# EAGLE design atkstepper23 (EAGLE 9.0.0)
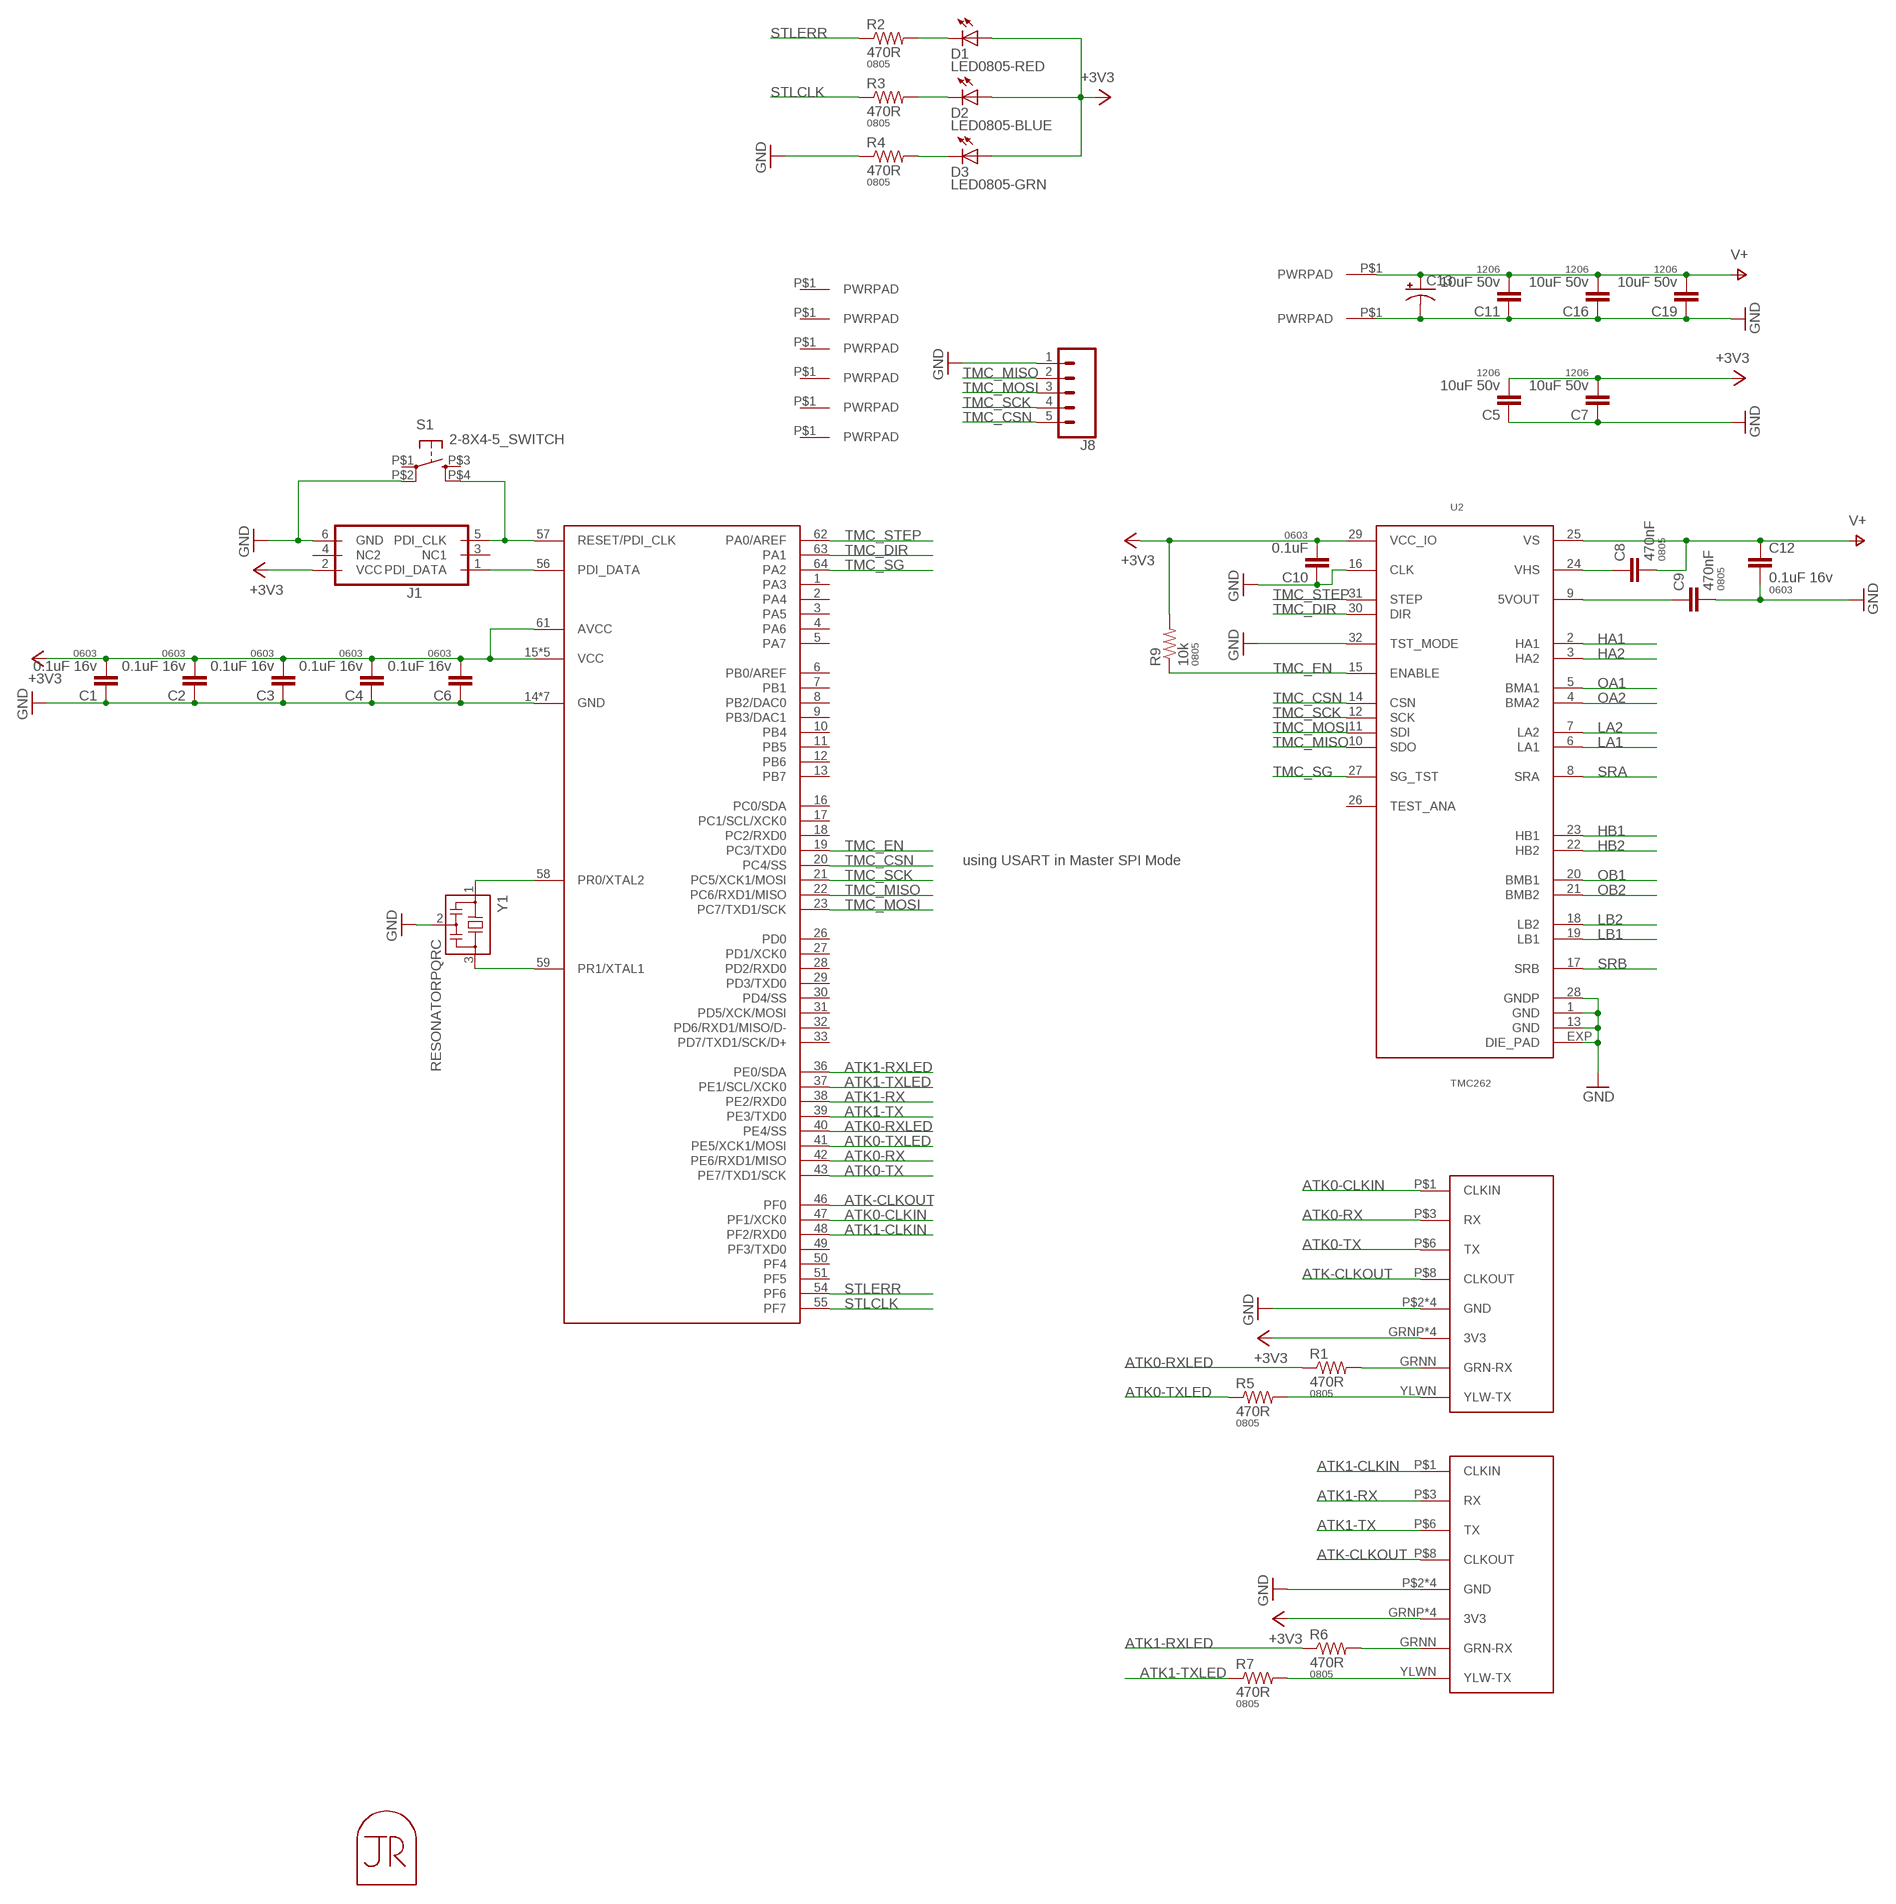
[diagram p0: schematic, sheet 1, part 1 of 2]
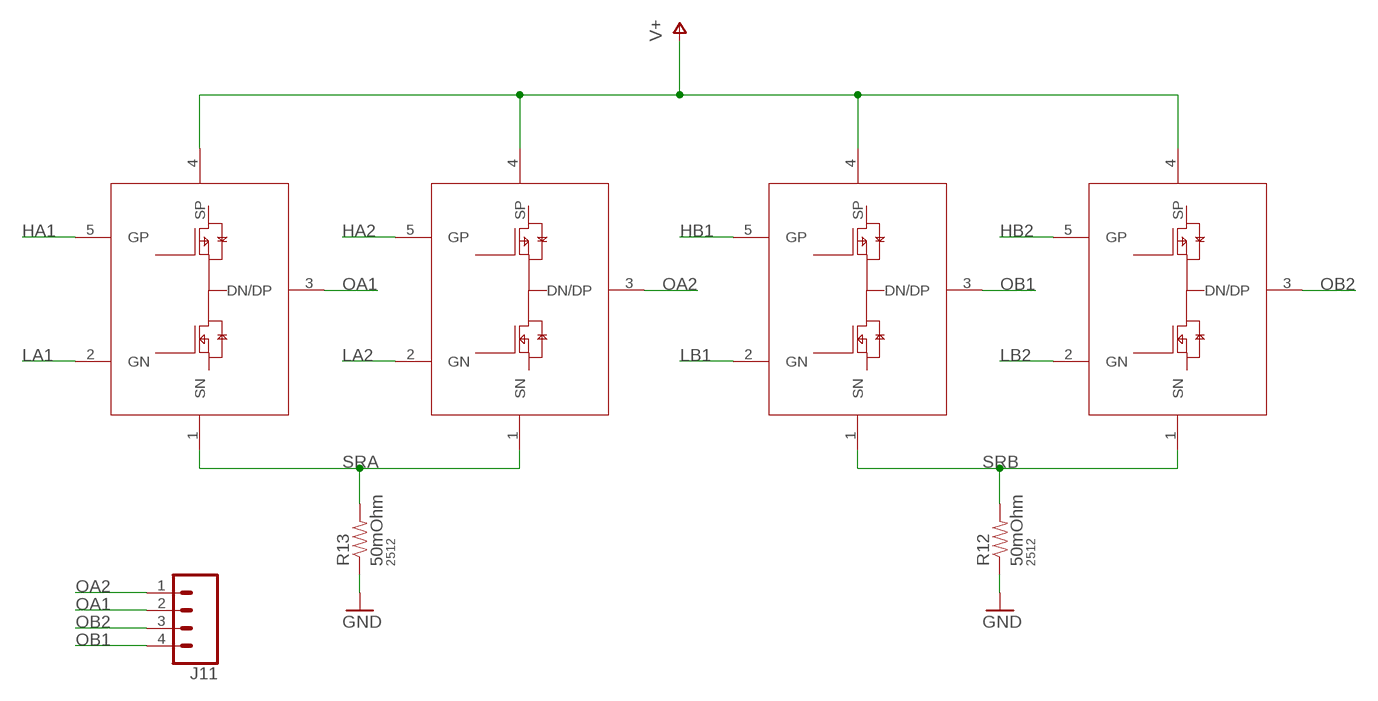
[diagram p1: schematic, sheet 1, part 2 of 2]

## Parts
C1  0.1uF 16v  CAP0603-CAP  [0603-CAP]
C2  0.1uF 16v  CAP0603-CAP  [0603-CAP]
C3  0.1uF 16v  CAP0603-CAP  [0603-CAP]
C4  0.1uF 16v  CAP0603-CAP  [0603-CAP]
C5  10uF 50v  CAP1206  [1206]
C6  0.1uF 16v  CAP0603-CAP  [0603-CAP]
C7  10uF 50v  CAP1206  [1206]
C8  470nF  CAP0805  [0805]
C9  470nF  CAP0805  [0805]
C10  0.1uF  CAP0603-CAP  [0603-CAP]
C11  10uF 50v  CAP1206  [1206]
C12  0.1uF 16v  CAP0603-CAP  [0603-CAP]
C13  CAP-POL-6.6X6.6  [6.6X6.6-CAP]
C16  10uF 50v  CAP1206  [1206]
C19  10uF 50v  CAP1206  [1206]
D1  LED0805-RED  LED0805  [LED0805]
D2  LED0805-BLUE  LED0805  [LED0805]
D3  LED0805-GRN  LED0805  [LED0805]
J1  PDIFEMALE_SMD  [PDI_2X3_SMD]
J2  ATK-PHY  [RJ45-LED-RJE7318800XXX]
J3  ATK-PHY  [RJ45-LED-RJE7318800XXX]
J4  PWRPADM3-SKINNY  [PWRPAD_3-25MM-SKINNY]
J5  PWRPADM3-SKINNY  [PWRPAD_3-25MM-SKINNY]
J6  PWRPADM3-SKINNY  [PWRPAD_3-25MM-SKINNY]
J7  PWRPADM3-SKINNY  [PWRPAD_3-25MM-SKINNY]
J8  CONN_05NO_SILK  [1X05_NO_SILK]
J9  PWRPAD  [PWRPAD_M3-PEM-MOUNT]
J10  PWRPAD  [PWRPAD_M3-PEM-MOUNT]
J11  CONN_04LONGPADS  [1X04_LONGPADS]
J12  PWRPADM3-SKINNY  [PWRPAD_3-25MM-SKINNY]
J13  PWRPADM3-SKINNY  [PWRPAD_3-25MM-SKINNY]
MP1  JRTOMBSTONE  [JRTOMBSTONE]
Q1  PNPAIR-FDD8424H  [DPAK-5]
Q2  PNPAIR-FDD8424H  [DPAK-5]
Q3  PNPAIR-FDD8424H  [DPAK-5]
Q4  PNPAIR-FDD8424H  [DPAK-5]
R1  470R  RESISTOR0805-RES  [0805]
R2  470R  RESISTOR0805-RES  [0805]
R3  470R  RESISTOR0805-RES  [0805]
R4  470R  RESISTOR0805-RES  [0805]
R5  470R  RESISTOR0805-RES  [0805]
R6  470R  RESISTOR0805-RES  [0805]
R7  470R  RESISTOR0805-RES  [0805]
R9  10k  RESISTOR0805-RES  [0805]
R12  50mOhm  RESISTOR2512  [R2512]
R13  50mOhm  RESISTOR2512  [R2512]
S1  2-8X4-5_SWITCH  [TACT-SWITCH-KMR6]
U1  ATXMEGA_A3UQFN  [QFN-64-9X9MM]
U2  TMC262  [QFN32]
Y1  RESONATORPQRC  [RES_PRQC]

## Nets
+3V3: C1.2 C2.2 C3.2 C4.2 C5.2 C6.2 C7.2 C10.2 D1.1(A) D2.1(A) D3.1(A) J1.2(VCC) J2.GRNP(3V3) J2.P$4(3V3) J2.P$5(3V3) J2.YLWP(3V3) J3.GRNP(3V3) J3.P$4(3V3) J3.P$5(3V3) J3.YLWP(3V3) R9.2 U1.15(VCC) U1.25(VCC) U1.35(VCC) U1.45(VCC) U1.53(VCC) U1.61(AVCC) U2.29(VCC_IO)
ATK0-CLKIN: J2.P$1(CLKIN) U1.47(PF1/XCK0)
ATK0-RX: J2.P$3(RX) U1.42(PE6/RXD1/MISO)
ATK0-RXLED: R1.1 U1.40(PE4/SS)
ATK0-TX: J2.P$6(TX) U1.43(PE7/TXD1/SCK)
ATK0-TXLED: R5.1 U1.41(PE5/XCK1/MOSI)
ATK1-CLKIN: J3.P$1(CLKIN) U1.48(PF2/RXD0)
ATK1-RX: J3.P$3(RX) U1.38(PE2/RXD0)
ATK1-RXLED: R6.1 U1.36(PE0/SDA)
ATK1-TX: J3.P$6(TX) U1.39(PE3/TXD0)
ATK1-TXLED: R7.1 U1.37(PE1/SCL/XCK0)
ATK-CLKOUT: J2.P$8(CLKOUT) J3.P$8(CLKOUT) U1.46(PF0)
GND: C1.1 C2.1 C3.1 C4.1 C5.1 C6.1 C7.1 C9.2 C10.1 C11.1 C12.2 C13.- C16.1 C19.1 J1.6(GND) J2.P$2(GND) J2.P$7(GND) J2.SHDL1(GND) J2.SHDL2(GND) J3.P$2(GND) J3.P$7(GND) J3.SHDL1(GND) J3.SHDL2(GND) J8.1 J10.P$1(PWRPAD) R4.1 R12.1 R13.1 S1.P$2(P1) U1.14(GND) U1.24(GND) U1.34(GND) U1.44(GND) U1.52(GND) U1.60(GND) U1.P$1(GND) U2.1(GND) U2.13(GND) U2.16(CLK) U2.28(GNDP) U2.32(TST_MODE) U2.EXP(DIE_PAD) Y1.2
HA1: Q1.5(GP) U2.2(HA1)
HA2: Q2.5(GP) U2.3(HA2)
HB1: Q3.5(GP) U2.23(HB1)
HB2: Q4.5(GP) U2.22(HB2)
LA1: Q1.2(GN) U2.6(LA1)
LA2: Q2.2(GN) U2.7(LA2)
LB1: Q3.2(GN) U2.19(LB1)
LB2: Q4.2(GN) U2.18(LB2)
N$1: D3.2(C) R4.2
N$2: C8.1 U2.24(VHS)
N$3: C9.1 U2.9(5VOUT)
N$4: J1.5(PDI_CLK) S1.P$4(S1) U1.57(RESET/PDI_CLK)
N$5: D2.2(C) R3.2
N$6: D1.2(C) R2.2
N$7: U1.58(PR0/XTAL2) Y1.1
N$8: U1.59(PR1/XTAL1) Y1.3
N$10: J1.1(PDI_DATA) U1.56(PDI_DATA)
N$11: J3.GRNN(GRN-RX) R6.2
N$12: J3.YLWN(YLW-TX) R7.2
N$17: J2.GRNN(GRN-RX) R1.2
N$18: J2.YLWN(YLW-TX) R5.2
OA1: J11.2 Q1.3(DN/DP) U2.5(BMA1)
OA2: J11.1 Q2.3(DN/DP) U2.4(BMA2)
OB1: J11.4 Q3.3(DN/DP) U2.20(BMB1)
OB2: J11.3 Q4.3(DN/DP) U2.21(BMB2)
SRA: Q1.1(SN) Q2.1(SN) R13.2 U2.8(SRA)
SRB: Q3.1(SN) Q4.1(SN) R12.2 U2.17(SRB)
STLCLK: R3.1 U1.55(PF7)
STLERR: R2.1 U1.54(PF6)
TMC_CSN: J8.5 U1.20(PC4/SS) U2.14(CSN)
TMC_DIR: U1.63(PA1) U2.30(DIR)
TMC_EN: R9.1 U1.19(PC3/TXD0) U2.15(ENABLE)
TMC_MISO: J8.2 U1.22(PC6/RXD1/MISO) U2.10(SDO)
TMC_MOSI: J8.3 U1.23(PC7/TXD1/SCK) U2.11(SDI)
TMC_SCK: J8.4 U1.21(PC5/XCK1/MOSI) U2.12(SCK)
TMC_SG: U1.64(PA2) U2.27(SG_TST)
TMC_STEP: U1.62(PA0/AREF) U2.31(STEP)
V+: C8.2 C11.2 C12.1 C13.+ C16.2 C19.2 J9.P$1(PWRPAD) Q1.4(SP) Q2.4(SP) Q3.4(SP) Q4.4(SP) U2.25(VS)
Unconnected: J1.3(NC1) J1.4(NC2) J4.P$1(PWRPAD) J5.P$1(PWRPAD) J6.P$1(PWRPAD) J7.P$1(PWRPAD) J12.P$1(PWRPAD) J13.P$1(PWRPAD) S1.P$1(P) S1.P$3(S) U1.1(PA3) U1.2(PA4) U1.3(PA5) U1.4(PA6) U1.5(PA7) U1.6(PB0/AREF) U1.7(PB1) U1.8(PB2/DAC0) U1.9(PB3/DAC1) U1.10(PB4) U1.11(PB5) U1.12(PB6) U1.13(PB7) U1.16(PC0/SDA) U1.17(PC1/SCL/XCK0) U1.18(PC2/RXD0) U1.26(PD0) U1.27(PD1/XCK0) U1.28(PD2/RXD0) U1.29(PD3/TXD0) U1.30(PD4/SS) U1.31(PD5/XCK/MOSI) U1.32(PD6/RXD1/MISO/D-) U1.33(PD7/TXD1/SCK/D+) U1.49(PF3/TXD0) U1.50(PF4) U1.51(PF5) U2.26(TEST_ANA)

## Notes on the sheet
- using USART in Master SPI Mode

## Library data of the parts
C1-C4 C6 C10 C12 = borkedlabs-passives:CAP: Capacitor; PACKAGE: 0603
C5 C7 C11 C16 C19 = borkedlabs-passives:CAP: Capacitor; PACKAGE: 1206
C8 C9 = borkedlabs-passives:CAP: Capacitor; PACKAGE: 0805
C13 = borkedlabs-passives:CAP-POL
D1-D3 = lights:LED: LED
J1 = microcontrollers:PDI: Multi connection point. Often used as Generic Header-pin footprint for 0.1 inch spaced/style header connections You can populate with any combo of single row headers, but if you'd like an exact match, check these: Header - 2x3 (Male, 0.1") (PRT-12807) Header - 2x3 (Female, 0.1") (PRT-13010) 2x3 Pin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; PROD_ID: CONN-11290
J2 J3 = connector:ATK-PHY
J4-J7 J9 J10 J12 J13 = power:PWRPAD
J8 = SparkFun-Connectors:CONN_05: Multi connection point. Often used as Generic Header-pin footprint for 0.1 inch spaced/style header connections On any of the 0.1 inch spaced packages, you can populate with these: Break Away Headers - Straight (PRT-00116) Break Away Male Headers - Right Angle (PRT-00553) Female Headers (PRT-00115)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
J11 = SparkFun-Connectors:CONN_04: Multi connection point. Often used as Generic Header-pin footprint for 0.1 inch spaced/style header connections On any of the 0.1 inch spaced packages, you can populate with these: Break Away Headers - Straight (PRT-00116) Break Away Male Headers - Right Angle (PRT-00553) Female Headers (PRT-00115)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; PROD_ID: CONN-09696
MP1 = connector:JRTOMBSTONE
Q1-Q4 = power:PNPAIR-FDD8424H
R1-R7 R9 = borkedlabs-passives:RESISTOR: Resistor; PACKAGE: 0805
R12 R13 = borkedlabs-passives:RESISTOR: Resistor; PACKAGE: 2512
S1 = fab:2-8X4-5_SWITCH
U1 = microcontrollers:ATXMEGA_A3U
U2 = power:TMC262
Y1 = passives:RESONATOR

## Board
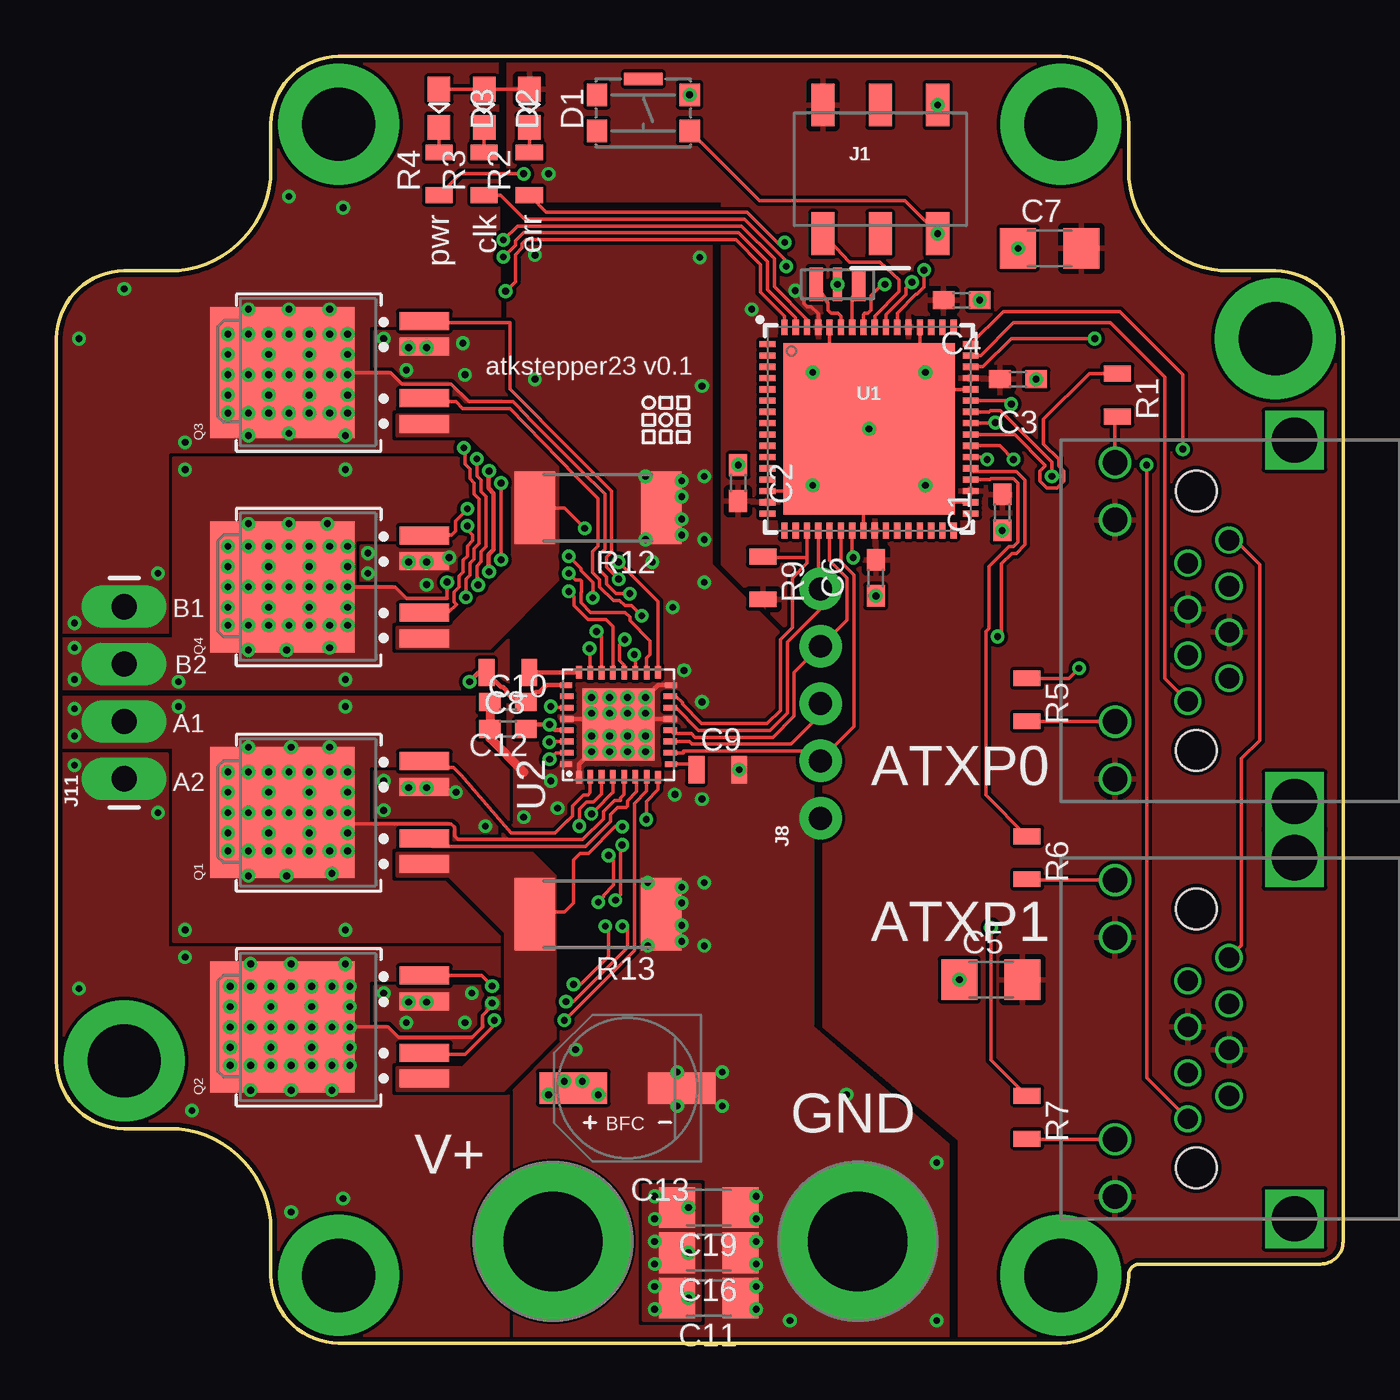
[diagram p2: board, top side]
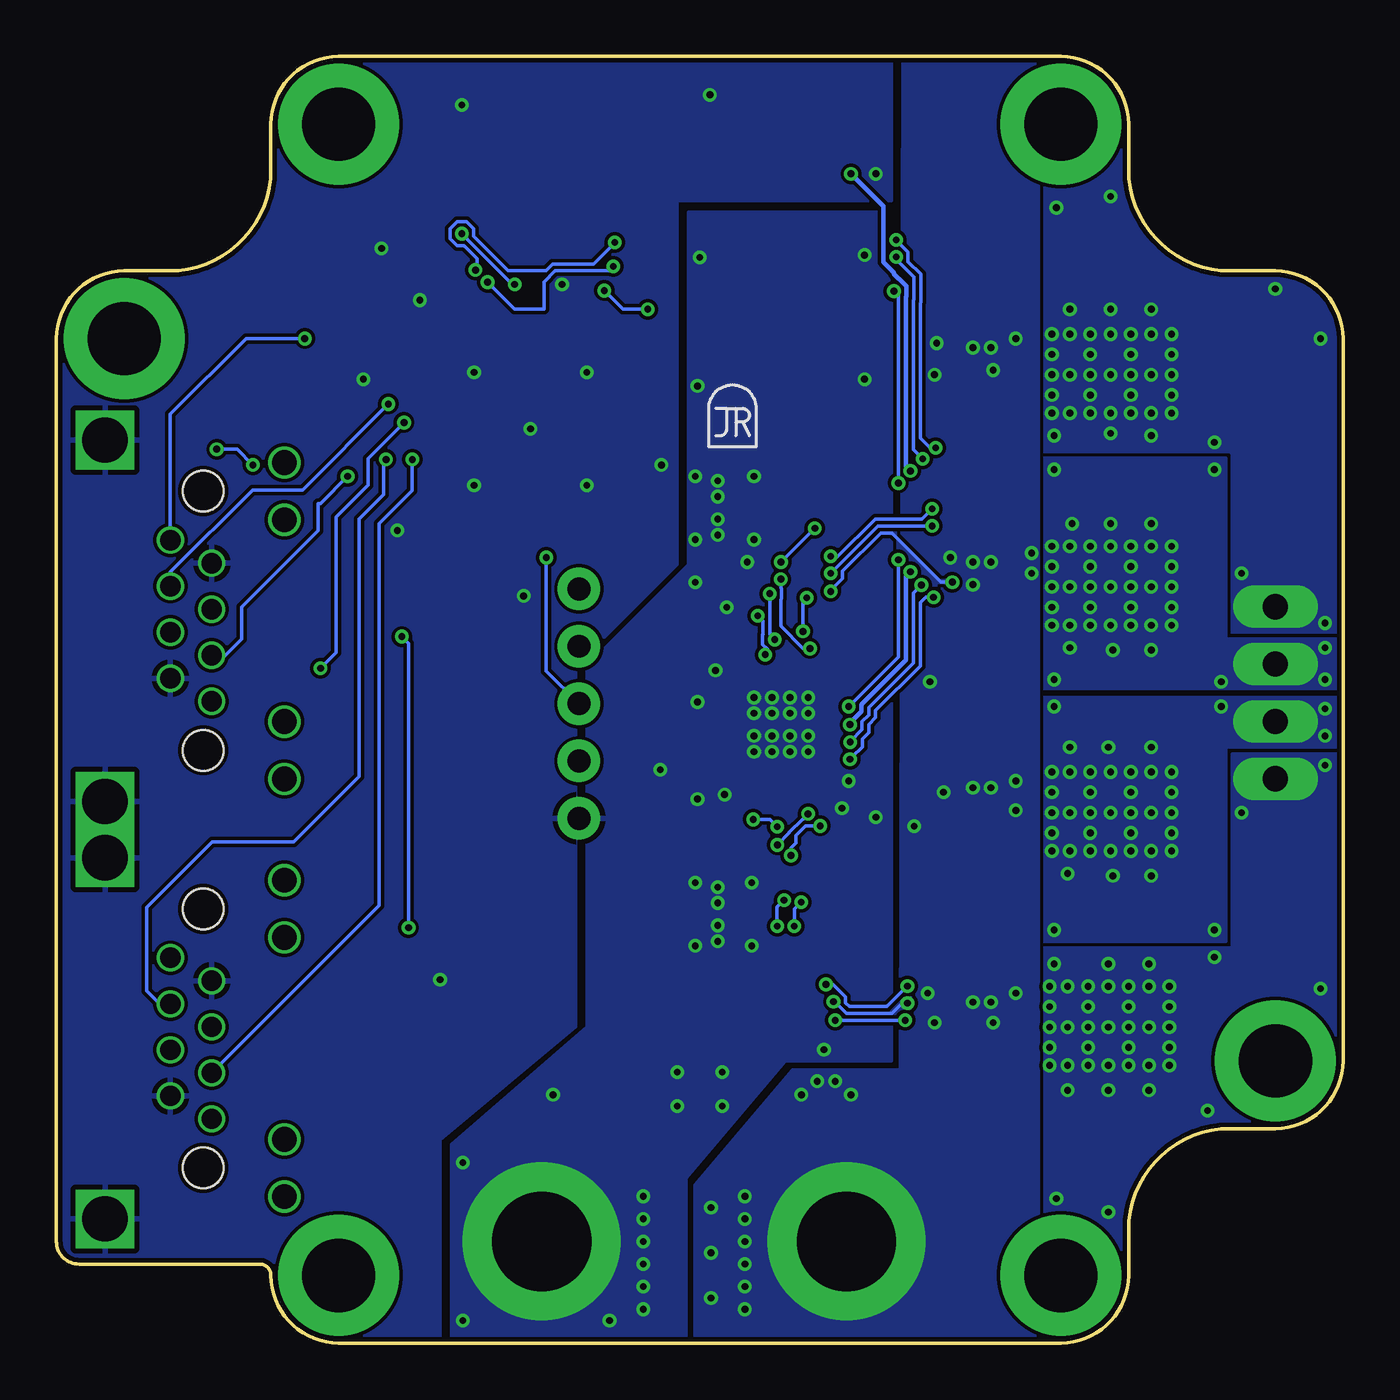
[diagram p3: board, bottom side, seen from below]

Size 57 x 57 mm. Coordinates in mm from the lower left corner, seen from the top.
Outline: 44.5,0 12.5,0 arc-90 9.5,3 9.5,5 arc90 5,9.5 3,9.5 arc-90 0,12.5 0,44.5 arc-90 3,47.5 5,47.5 arc90 9.5,52 9.5,54 arc-90 12.5,57 44.5,57 arc-90 47.5,54 47.5,52 arc90 52,47.5 54,47.5 arc-90 57,44.5 57,4.5 arc-90 56,3.5 48,3.5 arc90 47.5,3 arc-90 44.5,0
Copper layers (1*16): Top 0.035mm / dielectric 1.5mm / Bottom 0.035mm
Design rules "default *": minimum track width 6mil, minimum drill 0.3mm, track to track 6mil, track to pad 6mil, pad to pad 6mil, via to via 6mil, smd to smd 6mil, copper to edge 8mil, drill to drill 8mil, minimum pad ring 6mil, minimum via ring 6mil, stop-mask expansion 4mil, vias tented up to drill 27mil, thermal gap 9mil

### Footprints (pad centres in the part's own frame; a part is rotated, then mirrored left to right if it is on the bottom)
0603-CAP = smd 0.96 x 0.8: 1 -0.8,0; 2 0.8,0
1206 = smd 1.6 x 1.8: 1 -1.4,0; 2 1.4,0
0805 = smd 0.7 x 1.2: 1 -0.95,0; 2 0.95,0
6.6X6.6-CAP = smd 3 x 1.4: + 2.4,0; - -2.4,0
LED0805 = smd 1.1 x 1: 1 -0.85,0; 2 0.85,0
PDI_2X3_SMD = smd 1.02 x 1.9: 1 -2.54,-2.85; 2 -2.54,2.85; 3 0,-2.85; 4 0,2.85; 5 2.54,-2.85; 6 2.54,2.85
RJ45-LED-RJE7318800XXX = drill 1.1: GRNN 7.01,3.6; GRNP 4.47,3.6; YLWN -4.47,3.6; YLWP -7.01,3.6 | drill 0.9: P$1 -3.57,0.38; P$2 -2.55,-1.45; P$3 -1.53,0.38; P$4 -0.51,-1.45; P$5 0.51,0.38; P$6 1.53,-1.45; P$7 2.55,0.38; P$8 3.57,-1.45 | drill 2 square: SHDL1 -8,-4.35; SHDL2 8,-4.35 | hole 1.8: -5.74,0; 5.74,0
PWRPAD_3-25MM-SKINNY = drill 3.25 pad 5.35: P$1 0,0
1X05_NO_SILK = drill 1.016 pad 1.88: 1 0,0; 2 2.54,0; 3 5.08,0; 4 7.62,0; 5 10.16,0
PWRPAD_M3-PEM-MOUNT = drill 4.4 pad 7: P$1 0,0
1X04_LONGPADS = drill 1.118 pad 1.88 long: 1 0,0; 2 2.54,0; 3 5.08,0; 4 7.62,0
DPAK-5 = smd 0.8 x 2.2: 1 -2.28,-5.3; 2 -1.14,-5.3; 4 1.14,-5.3; 5 2.28,-5.3 | smd 5.8 x 6.4: 3 0,1
R2512 = smd 1.8 x 3.2: 1 -2.8,0; 2 2.8,0
TACT-SWITCH-KMR6 = smd 0.9 x 1: P$1 -2.05,0.8; P$2 2.05,0.8; P$3 -2.05,-0.8; P$4 2.05,-0.8 | smd 1.7 x 0.55: P$5 0,1.5
QFN-64-9X9MM = smd 0.7 x 0.275: 1 -4.5,3.75; 2 -4.5,3.25; 3 -4.5,2.75; 4 -4.5,2.25; 5 -4.5,1.75; 6 -4.5,1.25; 7 -4.5,0.75; 8 -4.5,0.25; 9 -4.5,-0.25; 10 -4.5,-0.75; 11 -4.5,-1.25; 12 -4.5,-1.75; 13 -4.5,-2.25; 14 -4.5,-2.75; 15 -4.5,-3.25; 16 -4.5,-3.75; 33 4.5,-3.75; 34 4.5,-3.25; 35 4.5,-2.75; 36 4.5,-2.25; 37 4.5,-1.75; 38 4.5,-1.25; 39 4.5,-0.75; 40 4.5,-0.25; 41 4.5,0.25; 42 4.5,0.75; 43 4.5,1.25; 44 4.5,1.75; 45 4.5,2.25; 46 4.5,2.75; 47 4.5,3.25; 48 4.5,3.75 | smd 0.275 x 0.7: 17 -3.75,-4.5; 18 -3.25,-4.5; 19 -2.75,-4.5; 20 -2.25,-4.5; 21 -1.75,-4.5; 22 -1.25,-4.5; 23 -0.75,-4.5; 24 -0.25,-4.5; 25 0.25,-4.5; 26 0.75,-4.5; 27 1.25,-4.5; 28 1.75,-4.5; 29 2.25,-4.5; 30 2.75,-4.5; 31 3.25,-4.5; 32 3.75,-4.5; 49 3.75,4.5; 50 3.25,4.5; 51 2.75,4.5; 52 2.25,4.5; 53 1.75,4.5; 54 1.25,4.5; 55 0.75,4.5; 56 0.25,4.5; 57 -0.25,4.5; 58 -0.75,4.5; 59 -1.25,4.5; 60 -1.75,4.5; 61 -2.25,4.5; 62 -2.75,4.5; 63 -3.25,4.5; 64 -3.75,4.5 | smd 7.6 x 7.6: P$1 0,0
QFN32 = smd 0.55 x 0.25: 1 -2.325,1.75; 8 -2.325,-1.75; 17 2.325,-1.75; 24 2.325,1.75 | smd 0.6 x 0.25: 2 -2.3,1.25; 3 -2.3,0.75; 4 -2.3,0.25; 5 -2.3,-0.25; 6 -2.3,-0.75; 7 -2.3,-1.25; 18 2.3,-1.25; 19 2.3,-0.75; 20 2.3,-0.25; 21 2.3,0.25; 22 2.3,0.75; 23 2.3,1.25 | smd 0.25 x 0.55: 9 -1.75,-2.325; 16 1.75,-2.325; 25 1.75,2.325; 32 -1.75,2.325 | smd 0.25 x 0.6: 10 -1.25,-2.3; 11 -0.75,-2.3; 12 -0.25,-2.3; 13 0.25,-2.3; 14 0.75,-2.3; 15 1.25,-2.3; 26 1.25,2.3; 27 0.75,2.3; 28 0.25,2.3; 29 -0.25,2.3; 30 -0.75,2.3; 31 -1.25,2.3 | smd 3.2 x 3.2: EXP 0,0
RES_PRQC = smd 0.6 x 1.5: 1 -0.95,0; 3 0.95,0 | smd 0.4 x 1.5: 2 0,0

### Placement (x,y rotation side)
C1  41.9,36.8 90 top
C2  30.2,38.1 270 top
C3  42.6,42.7 180 top
C4  40.1,46.2 180 top
C5  41.4,16.1 0 top
C6  36.3,33.9 90 top
C7  44,48.5 0 top
C8  20,29.7 180 top
C9  29.3,25.4 0 top
C10  20,27.2 0 top
C11  28.9,2 180 top
C12  20,28.4 180 top
C13  25.3,11.3 180 top
C16  28.9,4 180 top
C19  28.9,6 180 top
D1  20.95,54.7 270 top
D2  18.95,54.7 270 top
D3  16.95,54.7 270 top
J1  36.5,52 0 top
J2  50.5,32 90 top
J3  50.5,13.5 90 top
J4  12.5,3 180 top
J5  54,44.5 180 top
J6  44.5,3 180 top
J7  3,12.5 180 top
J8  33.85,23.25 90 top
J9  22,4.5 180 top
J10  35.5,4.5 180 top
J11  3,25 90 top
J12  12.5,54 180 top
J13  44.5,54 180 top
MP1  27,40.7 0 bottom
Q1  11,23.5 90 top
Q2  11,14 90 top
Q3  11,43 90 top
Q4  11,33.5 90 top
R1  47,42 270 top
R2  20.95,51.8 90 top
R3  18.95,51.8 90 top
R4  16.95,51.8 90 top
R5  43,28.5 270 top
R6  43,21.5 270 top
R7  43,10 270 top
R9  31.3,33.9 270 top
R12  24,37 180 top
R13  24,19 180 top
S1  26,54.5 0 top
U1  36,40.5 0 top
U2  24.9,27.4 90 top
U$5  [CBA-SILK-LOGO]  27,40.9 0 top
Y1  34.6,46.9 180 top

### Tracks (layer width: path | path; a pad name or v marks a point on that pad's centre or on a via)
+3V3  (via drill 0.3)
  Top 0.152: D1.1 D2.1 D3.1 | U1.61 33.75,45.6 33.43,45.92 33.26,45.92 33.12,46.05 33.12,46.23 v32.73,46.62
  Top 0.203: U2.29 22.09,27.15 v21.84,27.4 21,27.4 C10.2 | v19.16,34.16 19.16,34.45 19.14,34.47 19.14,34.93 19.37,35.16 19.37,37.64 19.14,37.87 19.14,38.33 19.16,38.35 v19.16,38.63
  Bottom 0.152: v32.73,46.62 31.9,45.8 v30.8,45.8
  Bottom 0.203: v21.84,27.4 21.84,27.47 21.34,27.97 21.34,28.29 19.37,30.26 19.37,33.96 v19.16,34.16 | v19.16,38.63 19.37,38.84 19.37,46.34 19.34,46.37 19.34,46.83 19.67,47.16 19.7,47.16 19.9,47.36 19.9,47.43 20.36,47.88 20.36,50.36 v21.8,51.8
  pour Top (rank 2): 20,58 20,50.6 29.5,50.6 29.5,34.5 34,30 34,14 40,9 40,-1 57.8,-0.8 57.8,58
ATK0-CLKIN
  Top 0.152: U1.47 40.95,43.75 42.4,45.2 46.7,45.2 49.1,42.8 49.1,29.45 J2.P$1
ATK0-RX  (via drill 0.3)
  Top 0.152: U1.42 41.32,41.25 41.38,41.31 41.82,41.31 44.1,39.03 v44.1,38.4
  Bottom 0.152: J2.P$3 49.53,30.47 48.8,31.2 48.8,32.6 45.4,36 45.4,37.2 45.3,37.2 v44.1,38.4
ATK0-RXLED
  Top 0.152: R1.1 45.75,42.95 43.73,40.93 43.73,39.83 44.41,39.16 44.41,38.85 44.63,38.62 44.63,38.18 44.32,37.87 43.88,37.87 43.57,38.18 43.57,38.62 43.8,38.85 43.8,38.91 42.45,40.25 U1.40
ATK0-TX  (via drill 0.3)
  Top 0.152: U1.43 42.15,41.75 v42.3,41.6
  Bottom 0.152: v42.3,41.6 46.1,37.8 48.3,37.8 51.95,34.15 J2.P$6
ATK0-TXLED  (via drill 0.3)
  Top 0.152: U1.41 41.57,40.75 v41.6,40.78 | v45.3,29.9 44.85,29.45 R5.1
  Bottom 0.152: v45.3,29.9 44.6,30.6 44.6,36.6 43.2,38 43.2,39.18 v41.6,40.78
ATK1-CLKIN  (via drill 0.3)
  Top 0.152: U1.48 41.95,45.7 47.1,45.7 49.9,42.9 v49.9,39.6 | v48.3,38.9 48.3,11.75 J3.P$1
  Bottom 0.152: v49.9,39.6 49,39.6 v48.3,38.9
ATK1-RX  (via drill 0.3)
  Top 0.152: U1.38 41.13,39.25 v41.24,39.14
  Bottom 0.152: v41.24,39.14 41.24,37.76 42.7,36.3 42.7,19.39 J3.P$3
ATK1-RXLED
  Top 0.152: U1.36 41.35,38.25 41.41,38.31 42.4,38.31 42.6,38.1 42.6,35.5 42.4,35.29 42.19,35.29 41.3,34.4 41.3,31.65 41.17,31.52 41.17,24.28 R6.1
ATK1-TX  (via drill 0.3)
  Top 0.152: U1.39 41.79,39.75 v42.4,39.14
  Bottom 0.152: v42.4,39.14 42.5,39.04 42.5,37.6 43.6,36.5 43.6,25.1 46.5,22.2 50.1,22.2 53,19.3 53,15.6 52.43,15.03 J3.P$6
ATK1-TXLED  (via drill 0.3)
  Top 0.152: U1.37 40.63,38.62 40.95,38.62 40.95,38.61 42.52,38.61 42.91,38.23 42.91,35.37 42.52,34.99 42.32,34.99 41.87,34.53 41.87,31.47 v41.7,31.3 | v41.4,18.4 41.4,12.55 R7.1
  Bottom 0.152: v41.7,31.3 41.4,31 v41.4,18.4
ATK-CLKOUT  (via drill 0.3)
  Top 0.152: U1.46 41.05,43.25 42.3,44.5 v46,44.5 | J2.P$8 52.23,35.57 53.3,34.5 53.3,26.7 52.5,25.9 52.5,17.62 J3.P$8
  Bottom 0.152: v46,44.5 48.6,44.5 51.95,41.15 J2.P$8
GND  (via drill 0.3)
  Top 0.152: R4.1 17.9,51.8 v20.7,51.8 | U1.60 34.25,42.25 35.9,40.6 | 35.9,40.6 U1.P$1 36.05,40.55 | U1.52 38.25,42.75 36.05,40.55 | U1.34 39.35,37.25 36.05,40.55 | U1.24 35.75,40.4 | 35.75,40.4 35.75,40.45 35.9,40.6 | U1.14 33.1,37.75 35.75,40.4 | U1.44 39.25,42.25 v38.5,43
  Top 0.203: U2.1 23.15,25.65 v23.7,26.2 | U2.13 26.35,27.65 v26.1,27.9 | U2.16 26.65,29.15 v26.1,28.6 | U2.28 23.45,27.65 v23.7,27.9
  Top 0.406: C12.2 C10.1 19.2,26.8 20.7,25.3
  other vias: 26.1,26.2 24.5,26.2 25.3,26.2 26.1,26.9 23.7,26.9 24.5,26.9 25.3,26.9 24.5,27.9 25.3,27.9 23.7,28.6 24.5,28.6 25.3,28.6 27.7,17.8 27.7,18.5 27.7,19.5 27.7,20.2 28.7,20.4 28.7,17.6 26.2,17.6 26.2,20.4 27.7,35.8 27.7,36.5 27.7,37.5 27.7,38.2 28.7,38.4 28.7,35.6 26.1,35.6 26.1,38.4 30.25,25.4 27.8,29.8 28.6,28.4 26.4,34.6 21.2,42.7 28.6,42.4 28.5,48.1 21.2,48.2 27.4,24.3 28.6,24.1 29.5,10.5 35,11 29.5,12 39,8 39,1 32.5,1 27.5,10.5 23,13 20.7,23.3 21.9,24.9 40.9,46.2 41.9,36 30.2,38.9 36.3,33.1 31,1.5 31,2.5 31,3.5 31,4.5 31,5.5 31,6.5 27.5,12 22.2,23.7 27.3,32.6 28.7,33.7 34.6,46.9 28.05,55.3 39.04,54.85 36,40.5 33.5,43 38.5,38 33.5,38 43.4,42.7 42.6,48.5 40,16.1
  pour Bottom: 29.1,-0.5 29.1,7.3 24.7,12.5 20,12.5 20,50.1 29,50.1 29,34.5 33.5,30 33.5,14 39.5,8.8 39.5,-0.5
  pour Top (no thermals): 25.8,35.3 29,35.3 29,38.7 25.8,38.7
  pour Top (no thermals): 25.8,17.3 29,17.3 29,20.7 25.8,20.7
  pour Bottom: 29.5,57.6 20,57.6 20,50.6 29.5,50.6 29.5,34.5 34,30 34,14 40,9 40,-0.5 57.5,-0.5 57.5,57.5
  pour Top (rank 6, no thermals): 39.5,-1 39.5,8.8 33.5,14 33.5,30 29,34.5 29,50.1 20,50.1 20,-1
HA1
  Top 0.152: Q1.5 16.58,25.5 17.6,25.5 17.93,25.17 20.13,22.61 22.1,22.61 22.64,23.14 22.64,23.13 22.86,23.36 22.86,23.79 23.36,24.28 23.54,24.28 23.65,24.39 U2.2
HA2  (via drill 0.3)
  Top 0.152: Q2.5 18.83,16.28 v19.3,15.81 | v22.91,15.89 23.23,15.89 24.47,17.13 24.47,18.31 v24.31,18.47 | v24.01,19.53 24.23,19.76 24.23,19.84 24.69,20.29 24.69,21.37 v24.46,21.6 | v23.17,22.91 23.17,23.66 23.48,23.98 23.8,23.98 24.15,24.32 U2.3
  Bottom 0.152: v19.3,15.81 20.2,14.91 21.87,14.91 22.04,15.08 22.04,15.35 22.59,15.89 v22.91,15.89 | v24.31,18.47 24.31,19.23 v24.01,19.53 | v24.46,21.6 24.46,21.94 24.23,22.16 24.23,22.48 23.81,22.91 v23.17,22.91
HB1  (via drill 0.3)
  Top 0.152: Q3.5 16.38,45.2 20.1,45.2 20.1,42.27 20.44,41.93 20.44,41.92 20.54,41.83 21.45,40.92 21.45,40.89 24.6,37.74 24.6,35.05 | v24.91,33.84 24.37,34.38 24.37,34.82 24.6,35.05 | 24.6,35.05 | U2.23 23.65,30.74 v23.62,30.77
  Bottom 0.152: v24.91,33.84 24.91,33.46 24.87,33.42 24.87,32.98 24.91,32.94 24.91,31.75 23.92,30.77 v23.62,30.77
HB2  (via drill 0.3)
  Top 0.152: Q4.5 16.32,35.8 17.5,35.8 17.67,35.97 17.67,36.42 v18.2,36.95 v18.2,36.96 | v22.7,34.86 v22.7,34.85 23.23,34.32 23.23,34.23 23.76,33.69 v23.76,33.02 | v23.93,31.53 24.15,31.31 U2.22
  Bottom 0.152: v18.2,36.96 18.66,36.51 20.73,36.51 22.42,34.82 22.66,34.82 v22.7,34.86 | v23.93,31.53 23.93,32.85 v23.76,33.02
LA1
  Top 0.152: U2.6 25.7,25.05 25.7,24.43 25.3,24.03 25.3,23.8 25.23,23.73 24.85,23.73 24.54,23.42 24.54,23.1 23.44,22 16.66,22 Q1.2
LA2  (via drill 0.3)
  Top 0.152: Q2.2 17.4,12.8 18.1,12.8 19.4,14.1 v19.4,14.3 | v22.5,14.3 25.6,17.4 25.6,23.9 26.15,24.45 U2.7
  Bottom 0.152: v19.4,14.3 v22.5,14.3
LB1  (via drill 0.3)
  Top 0.152: Q3.2 16.46,41.7 17.7,41.7 18,41.4 20.1,41.4 23,38.4 23.99,37.41 23.99,35.3 23.76,35.07 23.76,34.13 24.07,33.82 24.07,33.5 24.67,32.9 24.95,32.9 25.18,32.67 25.48,32.67 v25.93,32.22 | U2.19 25.65,30.45 v25.6,30.5
  Bottom 0.152: v25.6,30.5 25.5,30.6 25.5,30.74 25.71,30.95 25.71,31.39 25.7,31.4 25.7,31.99 v25.93,32.22
LB2  (via drill 0.3)
  Top 0.152: Q4.2 17.36,32.36 17.72,32.72 17.61,32.82 17.61,33.26 17.84,33.49 17.84,33.97 18.02,34.16 18.02,34.69 18.2,34.87 18.2,35.32 18.43,35.55 18.43,35.8 18.2,36.03 v18.2,36.2 | U2.18 26.15,30.35 26.3,30.5 26.3,31.1 25.4,32 25.4,32.16 25.2,32.36 23.67,32.36 23.23,32.8 23.23,33.24 23.26,33.27 23.26,33.76 23.23,33.8 23,33.8 v22.7,34.1
  Bottom 0.152: v18.2,36.2 20.6,36.2 v22.7,34.1
N$1
  Top 0.152: D3.2 R4.2
N$2
  Top 0.203: U2.24 23.12,29.7 C8.1
N$3
  Top 0.152: U2.9 28.35,25.65 C9.1
N$4  (via drill 0.3)
  Top 0.152: U1.57 35.75,45.57 35.8,45.62 35.95,45.62 36.08,45.76 36.08,46.4 36.58,46.9 v36.7,46.9 | S1.P$4 31.15,50.6 37.59,50.6 J1.5
  Bottom 0.152: J1.5 38.81,48.92 38.81,48.91 36.8,46.9 v36.7,46.9
  other vias: 39.04,49.15
N$5
  Top 0.152: D2.2 R3.2
N$6
  Top 0.152: D1.2 R2.2
N$7
  Top 0.152: U1.58 35.25,46.3 Y1.1
N$8
  Top 0.152: U1.59 34.75,45.5 34.63,45.62 34.3,45.62 34.17,45.76 34.17,46.08 Y1.3
N$10
  Top 0.152: J1.1 35.13,47.88 36.47,47.88 37.33,47.12 37.33,46.58 36.25,45.5 U1.56
N$11
  Top 0.152: J3.GRNN 43.04,20.51 R6.2
N$12
  Top 0.152: J3.YLWN 43.02,9.03 R7.2
N$17
  Top 0.152: J2.GRNN 46.9,40.95 R1.2
N$18
  Top 0.152: J2.YLWN 43.02,27.53 R5.2
OA1  (via drill 0.3)
  Top 0.152: U2.5 25.15,24.31 24.99,24.15 24.99,24.04 24.72,24.04 24.23,23.55 24.23,23.23 23.31,22.3 17.8,22.3 17.63,22.48 17.63,22.86 17.5,22.99 10.51,22.99 Q1.3
  other vias: 7.6,21.8 7.6,22.6 7.6,23.5 7.6,24.4 7.6,25.3 12.9,21.8 12.9,22.6 12.9,23.5 12.9,24.4 12.9,25.3 12.1,21.8 12.2,20.8 12.1,23.5 12.1,26.4 12.1,25.3 11.2,21.8 11.2,22.6 11.2,23.5 11.2,24.4 11.2,25.3 10.3,21.8 10.2,20.7 10.3,23.5 10.4,26.4 10.3,25.3 9.4,21.8 9.4,22.6 9.4,23.5 9.4,24.4 9.4,25.3 8.5,21.8 8.5,20.7 8.5,23.5 8.5,26.4 8.5,25.3 12.8,28.2 5.4,28.2 0.8,28.1 0.8,26.9 5.7,18.3 12.8,18.3
  pour Top (rank 2, no thermals): -0.3,28.6 20,28.6 20,17.8 5.2,17.8 5.2,26.4 -0.3,26.4
  pour Bottom (rank 2, no thermals): -0.3,28.6 20,28.6 20,17.8 5.2,17.8 5.2,26.4 -0.3,26.4
OA2  (via drill 0.3)
  Top 0.152: Q2.3 14.7,14 15.16,13.54 18.41,13.54 18.87,14 18.87,14.52 19.3,14.95 v19.3,15.06 | v22.57,15.12 22.89,15.12 25.3,17.53 25.3,18.4 25.23,18.47 v25.07,18.47 | v24.76,19.62 24.99,19.85 24.99,22 v25.06,22.07 | U2.4 24.65,24.39 24.6,24.34 | 24.6,24.34 | 23.93,23.67 | 23.93,23.67 v23.7,23.45 | 24.6,24.34 23.93,23.67
  Bottom 0.152: v19.3,15.06 19.54,15.06 20,14.61 22,14.61 22.52,15.12 v22.57,15.12 | v25.07,18.47 25.07,19.32 v24.76,19.62 | v23.7,23.45 23.7,23.43 23.91,23.22 23.93,23.22 24.54,22.61 24.54,22.59 v25.06,22.07
  other vias: 7.7,12.3 7.7,13.1 7.7,14 7.7,14.9 7.7,15.8 13,12.3 13,13.1 13,14 13,14.9 13,15.8 12.2,12.3 12.2,11.2 12.2,14 5.7,17.1 12.2,15.8 11.3,12.3 11.3,13.1 11.3,14 11.3,14.9 11.3,15.8 10.4,12.3 10.4,11.2 10.4,14 10.4,16.8 10.4,15.8 9.5,12.3 9.5,13.1 9.5,14 9.5,14.9 9.5,15.8 8.6,12.3 8.6,11.2 8.6,14 8.6,16.8 8.6,15.8 0.8,25.6 4.5,23.5 1,15.7 6,10.3 12.8,16.8 12.7,6.4 10.4,5.8
  pour Top (rank 4, no thermals): -0.3,26.1 4.9,26.1 4.9,17.5 20,17.5 20,-1.5 -0.3,-1.5
  pour Bottom (rank 4, no thermals): -0.3,26.1 4.9,26.1 4.9,17.5 20,17.5 20,-1.1 -0.3,-1.1
OB1  (via drill 0.3)
  Top 0.152: Q3.3 14.8,43 15.31,42.49 17.5,42.49 18.28,41.7 19.98,41.7 19.98,41.71 20.1,41.7 20.23,41.7 20.32,41.61 20.41,41.53 20.41,41.52 21.05,40.85 23.2,38.71 | 23.2,38.71 23.2,38.7 | 23.2,38.71 24.3,37.61 24.3,35.18 24.06,34.95 24.06,34.25 24.38,33.94 24.38,33.62 24.8,33.2 v25.4,33.2 | U2.20 25.15,30.05 24.95,30.25 24.95,30.94 v25.18,31.17
  Bottom 0.152: v25.4,33.2 25.4,31.39 v25.18,31.17
  other vias: 7.6,41.2 7.6,42 7.6,42.9 7.6,43.8 7.6,44.7 12.9,41.2 12.9,42 12.9,42.9 12.9,43.8 12.9,44.7 12.1,41.2 12.1,42.9 12.1,45.8 12.1,44.7 11.2,41.2 11.2,42 11.2,42.9 11.2,43.8 11.2,44.7 10.3,41.2 10.3,40.3 10.3,42.9 10.3,45.8 10.3,44.7 9.4,41.2 9.4,42 9.4,42.9 9.4,43.8 9.4,44.7 8.5,41.2 8.5,40.2 8.5,42.9 8.5,45.8 8.5,44.7 0.8,31.9 4.5,34.1 5.7,39.9 1,44.5 3,46.7 12.8,40.2 12.7,50.3 10.3,50.8
  pour Top (rank 3, no thermals): -0.3,31.5 5,31.5 5,39.5 19.7,39.5 19.5,58.3 -0.5,58.3
  pour Bottom (rank 3, no thermals): -0.3,31.5 5,31.5 5,39.5 20,39.5 20,57.7 -0.3,57.7
OB2  (via drill 0.3)
  Top 0.152: Q4.3 15,33.5 15.51,32.99 17.3,32.99 v17.3,33.7 v17.31,33.71 | v22.7,33.3 22.93,33.07 22.93,32.67 23.54,32.06 24.34,32.06 24.65,31.75 U2.21
  Bottom 0.152: v17.31,33.71 17.81,33.71 20,35.9 20.47,35.9 22.17,34.2 22.17,33.88 22.7,33.35 v22.7,33.3
  other vias: 7.6,31.8 7.6,32.6 7.6,33.5 7.6,34.4 7.6,35.3 12.9,31.8 12.9,32.6 12.9,33.5 12.9,34.4 12.9,35.3 12.1,31.8 12.1,30.8 12.1,33.5 12,36.3 12.1,35.3 11.2,31.8 11.2,32.6 11.2,33.5 11.2,34.4 11.2,35.3 10.3,31.8 10.2,30.7 10.3,33.5 10.3,36.3 10.3,35.3 9.4,31.8 9.4,32.6 9.4,33.5 9.4,34.4 9.4,35.3 8.5,31.8 8.5,30.7 8.5,33.5 8.5,36.3 8.5,35.3 5.7,38.7 0.8,29.4 0.8,30.8 5.4,29.3 12.8,29.4 12.8,38.7
  pour Top (rank 2, no thermals): -0.3,29 20,29 20,39.2 5.2,39.2 5.2,31.2 -0.3,31.2
  pour Bottom (rank 2, no thermals): -0.3,29 20,29 20,39.2 5.2,39.2 5.2,31.2 -0.3,31.2
SRA  (via drill 0.3)
  Top 0.152: R13.2 21.3,19.1 22.5,19.1 22.9,19.5 22.9,21.4 23.2,21.7 23.56,21.7 24.75,22.88 v25.07,22.88 | v26.13,23.2 26.13,24 26.65,24.52 U2.8
  Bottom 0.152: v25.07,22.88 25.39,23.2 v26.13,23.2
  pour Top (no thermals): 15.1,12.2 18,12.2 19.9,14.1 19.9,18.2 17.4,20.7 15.1,20.7 15.1,21.7 21.1,21.7 22.1,20.7 22.1,13.5 19.8,11.2 15.1,11.2
SRB  (via drill 0.3)
  Top 0.152: R12.2 22.5,37 v23.4,36.1 | v24.9,34.6 26.65,32.85 U2.17
  Bottom 0.152: v23.4,36.1 v24.9,34.6
  pour Top (no thermals): 15.1,31.7 17.4,31.7 20.2,34.5 20.2,38.3 18.3,40.2 15.1,40.2 15.1,41.1 19.9,41.1 22.2,38.8 22.2,33.8 19.2,30.8 15.1,30.8
STLCLK  (via drill 0.3)
  Top 0.152: R3.1 19.68,50.85 20.73,49.8 30.47,49.8 32.33,47.94 v32.33,47.7 | v37.9,47 37.64,46.74 37.64,46.45 36.75,45.56 U1.55
  Bottom 0.152: v32.33,47.7 32.53,47.5 34.9,47.5 35.4,47 35.4,45.8 36.7,45.8 v37.9,47
STLERR  (via drill 0.3)
  Top 0.152: R2.1 21.7,50.1 30.6,50.1 32.1,48.6 v32.26,48.76 | v38.44,47.53 38.44,46.78 38.12,46.47 38.09,46.47 37.25,45.63 U1.54
  Bottom 0.152: v32.26,48.76 33.22,47.8 35.03,47.8 35.32,47.52 36.98,47.52 38.51,49.04 38.51,49.37 38.82,49.68 39.26,49.68 39.57,49.37 39.57,48.93 39.26,48.62 38.95,48.62 38.37,48.03 38.37,47.6 v38.44,47.53
TMC_CSN
  Top 0.152: U2.14 27.45,28.15 28.45,27.14 31.61,27.14 32.38,27.91 32.38,31.05 33.85,32.52 J8.5 33.75,33.51 U1.20
TMC_DIR  (via drill 0.3)
  Top 0.152: U2.30 21.86,26.65 v21.84,26.62 | v18.68,33.58 18.68,33.9 18.63,33.95 18.63,34.43 18.81,34.61 18.81,35.07 19.04,35.29 19.04,37.51 18.81,37.73 18.81,38.24 18.63,38.41 v18.63,39.17 | v19.8,48.11 20.33,48.65 20.33,48.83 20.69,49.19 30.22,49.19 31.5,47.91 31.5,46.67 32.75,45.42 U1.63
  Bottom 0.152: v21.84,26.62 21.84,26.66 21.31,27.18 21.31,27.53 21.01,27.83 21.01,28.15 19.04,30.13 19.04,33.22 v18.68,33.58 | v18.63,39.17 19.04,39.58 19.04,46.21 19.01,46.23 19.01,47.22 19.8,48.01 v19.8,48.11
TMC_EN
  Top 0.152: U2.15 27.45,28.65 27.73,28.37 27.73,28.3 28.58,27.45 31.49,27.45 32.07,28.03 32.07,31.18 32.6,31.7 32.6,33.9 33.25,34.55 33.25,34.8 | 33.25,34.8 U1.19 | R9.1 31.35,34.8 33.25,34.8
TMC_MISO
  Top 0.152: U2.10 27.77,26.15 27.77,26.23 33.41,26.23 33.82,25.82 | 33.82,25.82 J8.2 | U1.22 34.75,34.59 35.32,34.02 35.32,27.32 33.82,25.82
TMC_MOSI  (via drill 0.3)
  Top 0.152: U2.11 28.05,26.65 28.17,26.53 32.53,26.53 33.85,27.85 J8.3 | U1.23 35.25,34.85 v35.3,34.8
  Bottom 0.152: v35.3,34.8 35.3,29.78 J8.3
TMC_SCK
  Top 0.152: U2.12 27.35,27 28.13,27 28.29,26.84 31.74,26.84 32.68,27.78 32.68,29.7 J8.4 35.02,32.04 35.02,33.89 34.25,34.66 U1.21
TMC_SG  (via drill 0.3)
  Top 0.152: U2.27 21.95,28.15 v21.9,28.2 | v19.7,34.7 v19.7,38.1 | v19.9,46.6 20.33,47.03 20.33,48.21 20.64,48.52 20.64,48.7 20.81,48.88 30.09,48.88 31.19,47.78 31.19,46.55 32.25,45.49 U1.64
  Bottom 0.152: v21.9,28.2 19.7,30.4 v19.7,34.7 | v19.7,38.1 19.7,46.4 v19.9,46.6
TMC_STEP  (via drill 0.3)
  Top 0.152: v18.14,33.04 18.14,33.84 18.33,34.03 18.33,34.56 18.51,34.74 18.51,35.19 18.73,35.42 18.73,37.38 18.51,37.61 18.51,38.11 18.33,38.29 18.33,38.72 18.1,38.95 18.1,39.6 v18.04,39.66 | v19.8,48.87 20.42,49.49 30.35,49.49 31.8,48.04 31.8,46.8 33.25,45.35 U1.62 | U2.31 22.13,26.15 v21.84,25.87
  Bottom 0.152: v21.84,25.87 21.62,26.09 21.61,26.09 21.41,26.3 21.4,26.3 21.3,26.4 21.3,26.76 21.01,27.05 21.01,27.41 20.71,27.71 20.71,28.03 18.73,30 18.73,32.8 18.49,33.04 v18.14,33.04 | v18.04,39.66 18.29,39.66 18.73,40.1 18.73,46.08 18.71,46.11 18.71,47.35 19.27,47.91 19.27,48.33 v19.8,48.87
V+  (via drill 0.3)
  Top 0.152: v22.5,11.6 22.6,11.6 C13.+
  Top 0.203: U2.25 21.71,29.15 21.41,28.85 21.25,28.85 C12.1 20.35,28.4 19.93,28.82 19.93,28.91 19.79,29.05 19.7,29.05 C8.2 18.7,29.7 v18.3,29.3
  other vias: 15.6,15.1 15.6,24.6 15.6,34.6 15.6,44.1 16.4,15.1 15.5,14.2 18.1,14.2 18.4,15.5 14.5,15.5 16.4,24.6 14.5,24.9 14.5,23.6 19,22.9 17.7,24.4 16.4,33.6 13.8,34.1 16.4,34.6 13.8,35 17.4,34.8 16.4,44.1 14.5,44.5 15.5,43.1 18.1,42.9 18,44.3 24,11 21.8,11 23.3,11.6 26.5,6.5 26.5,5.5 26.5,4.5 26.5,3.5 26.5,2.5 26.5,1.5 28,2 28,4 28,6
  pour Bottom: 13.5,-0.5 28.7,-0.5 28.7,7 24.4,12.1 19.6,12.1 19.5,57.5 13.5,57.5
  pour Top (rank 2, no thermals): 20,15.8 14.1,15.8 14.1,13.5 20,13.5
  pour Top (no thermals): 19.5,25.3 14.1,25.3 14.1,22.3 19.5,22.3
  pour Top (no thermals): 17.4,35.3 13.5,35.3 13.5,33.5 14.9,33.5 15.4,33 17.5,33 18.4,33.9 18.4,35.7 17.5,35.7 17.4,35.6
  pour Top (no thermals): 20.1,44.8 14.1,44.8 14.1,41.6 20.1,41.6
  pour Top (no thermals): 28.5,1 26,1 26,7 28.5,7

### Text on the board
tPlace: pwr | clk | err | atkstepper23 v0.1 | B1 | B2 | A1 | ATXP0 | A2 | ATXP1 | GND | V+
